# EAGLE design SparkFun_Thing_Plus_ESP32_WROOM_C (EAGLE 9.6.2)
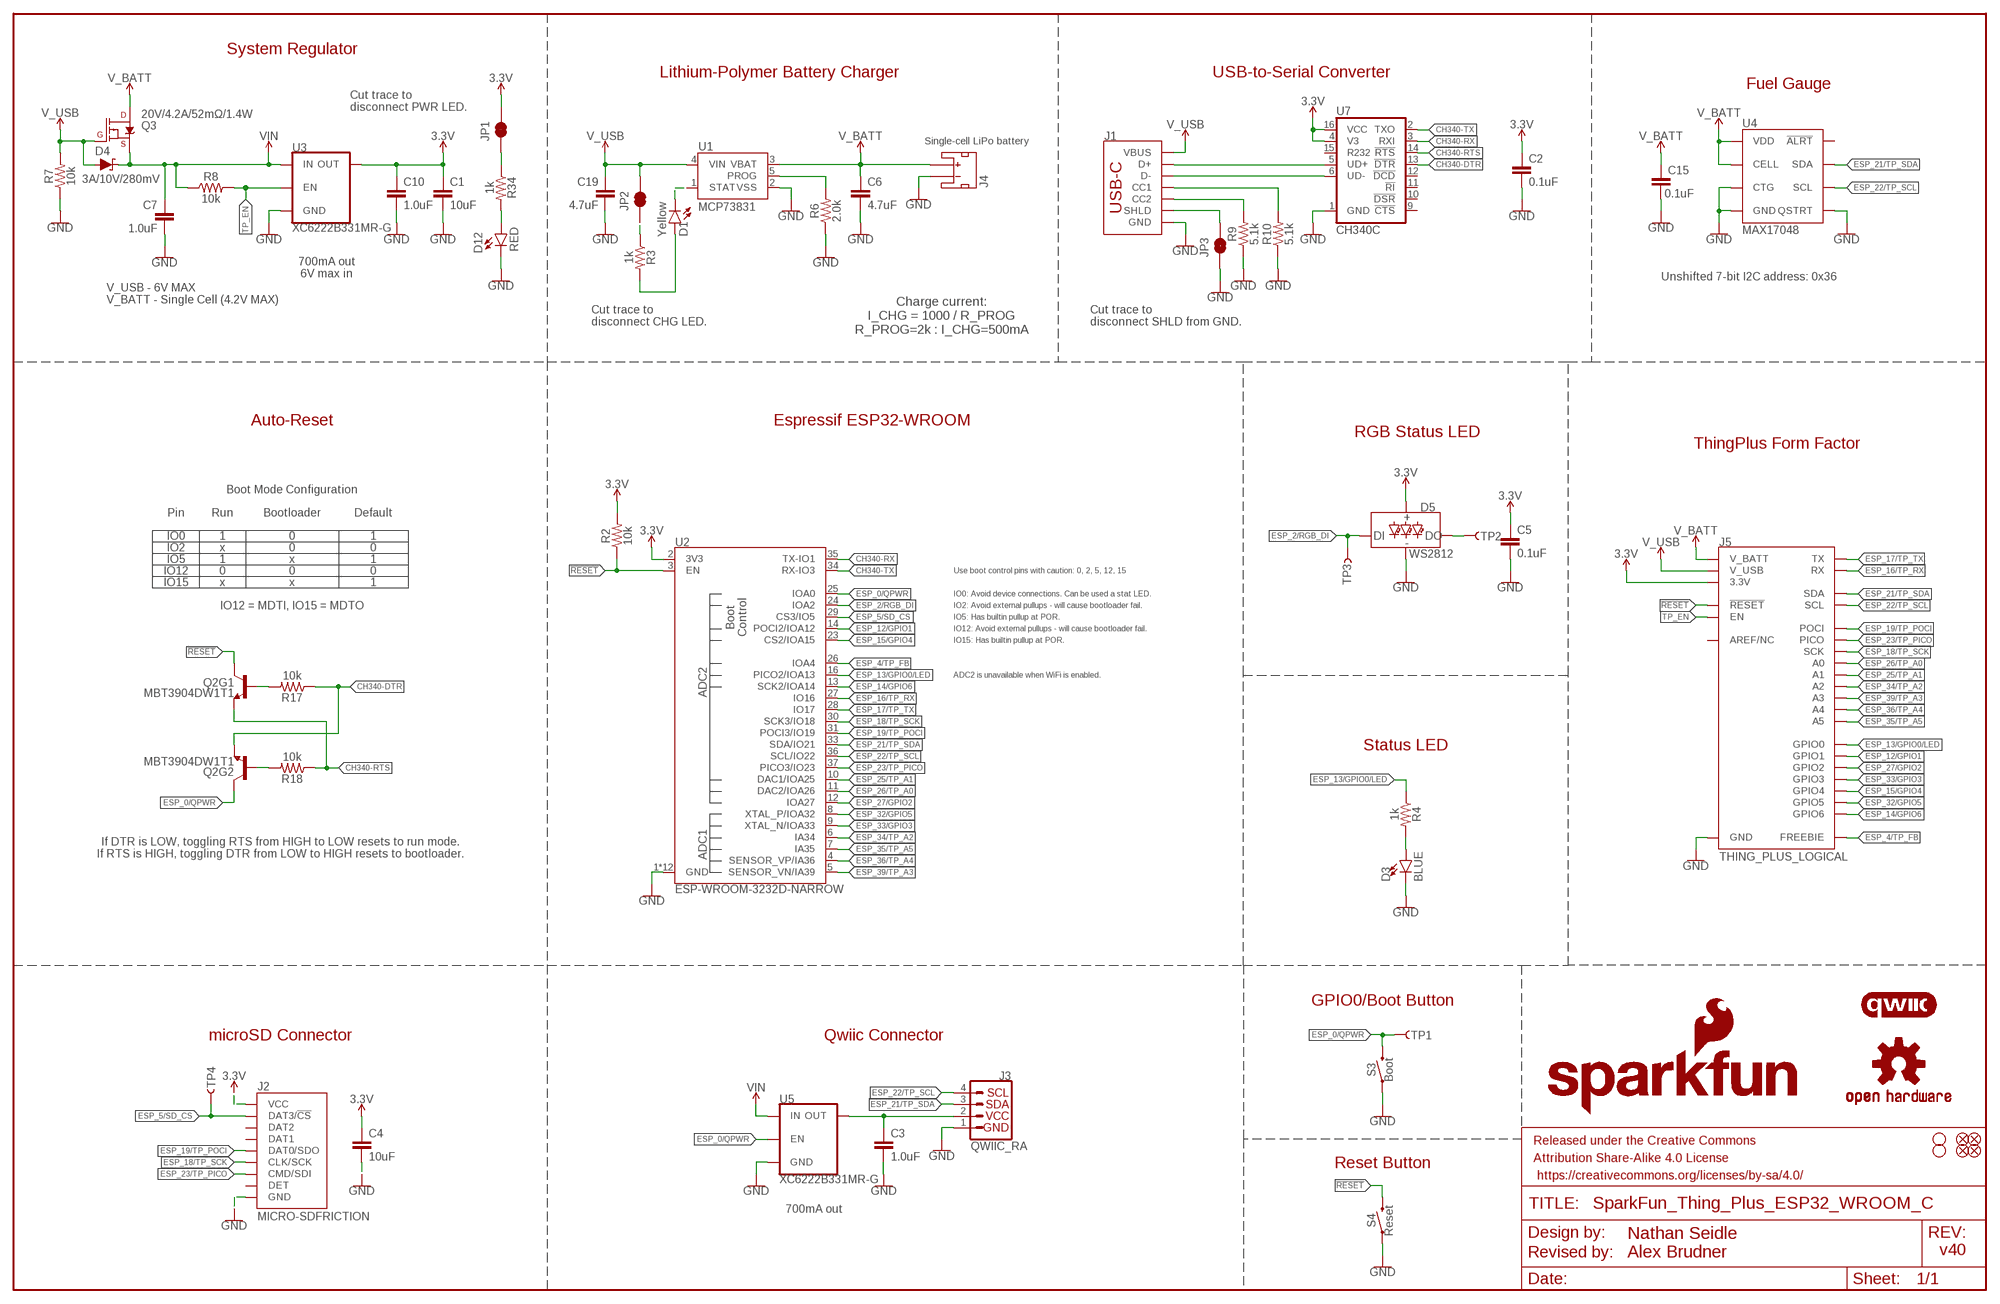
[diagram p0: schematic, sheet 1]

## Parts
C1  10uF  10UF-0402T-6.3V-20%  [0402-TIGHT]
C2  0.1uF  0.1UF-0402T-6.3V-10%-X7R  [0402-TIGHT]
C3  1.0uF  1.0UF-0402T-16V-10%  [0402-TIGHT]
C4  10uF  10UF-0402T-6.3V-20%  [0402-TIGHT]
C5  0.1uF  0.1UF-0402T-6.3V-10%-X7R  [0402-TIGHT]
C6  4.7uF  4.7UF-0402_TIGHT-6.3V-20%-X5R  [0402-TIGHT]
C7  1.0uF  1.0UF-0402T-16V-10%  [0402-TIGHT]
C10  1.0uF  1.0UF-0402T-16V-10%  [0402-TIGHT]
C15  0.1uF  0.1UF-0402T-16V-10%  [0402-TIGHT]
C19  4.7uF  4.7UF-0603-35V-(20%)  [0603]
D1  Yellow  LED-YELLOW0603  [LED-0603]
D3  BLUE  LED-BLUE0603  [LED-0603]
D4  3A/10V/280mV  DIODE-SCHOTTKY-BAT60A  [SOD-323]
D5  WS2812  WS2812_2020  [WS2812-2020]
D12  RED  LED-RED0603  [LED-0603]
FD1  FIDUCIALUFIDUCIAL  [FIDUCIAL-MICRO]
FD2  FIDUCIALUFIDUCIAL  [FIDUCIAL-MICRO]
FD3  FIDUCIALUFIDUCIAL  [FIDUCIAL-MICRO]
FD4  FIDUCIALUFIDUCIAL  [FIDUCIAL-MICRO]
FRAME1  FRAME-LEDGER  [CREATIVE_COMMONS]
H1  STAND-OFFTIGHT  [STAND-OFF-TIGHT]
H2  STAND-OFFTIGHT  [STAND-OFF-TIGHT]
J1  USB_C_2-LAYER_PADS  [USB-C-16P-2LAYER-PADS]
J2  MICRO-SDFRICTION  [MICROSD_TINY]
J3  QWIIC_RA  QWIIC_CONNECTORJS-1MM  [JST04_1MM_RA]
J4  JST_2MM_MALE  [JST-2-SMD]
J5  THING_PLUS_LOGICAL  [THING_PLUS]
JP1  JUMPER-SMT_2_NC_TRACE_SILK  [SMT-JUMPER_2_NC_TRACE_SILK]
JP2  JUMPER-SMT_2_NC_TRACE_SILK  [SMT-JUMPER_2_NC_TRACE_SILK]
JP3  JUMPER-SMT_2_NC_TRACE_SILK  [SMT-JUMPER_2_NC_TRACE_SILK]
LOGO1  SFE_LOGO_NAME_FLAME.1_INCH  [SFE_LOGO_NAME_FLAME_.1]
LOGO2  OSHW-LOGOMINI  [OSHW-LOGO-MINI]
LOGO4  QWIIC_LOGO_4MM  [QWIIC_4MM]
Q2  MBT3904DW1T1  TRANS_NPN_DUAL-MBT3904DW1T1  [SC70-6]
Q3  20V/4.2A/52mΩ/1.4W  MOSFET_PCH-DMG2305UX-7  [SOT23-3]
R2  10k  10KOHM-0402T-1/16W-1%  [0402-TIGHT]
R3  1k  1KOHM-0402T-1/16W-1%  [0402-TIGHT]
R4  1k  1KOHM-0402T-1/16W-1%  [0402-TIGHT]
R6  2.0k  2.0KOHM-0603-1/10W-5%  [0603]
R7  10k  10KOHM-0402T-1/16W-1%  [0402-TIGHT]
R8  10k  10KOHM-0402T-1/16W-1%  [0402-TIGHT]
R9  5.1k  5.1KOHM-0402T-1/16W-1%  [0402-TIGHT]
R10  5.1k  5.1KOHM-0402T-1/16W-1%  [0402-TIGHT]
R17  10k  10KOHM-0402T-1/16W-1%  [0402-TIGHT]
R18  10k  10KOHM-0402T-1/16W-1%  [0402-TIGHT]
R34  1k  1KOHM-0402T-1/16W-1%  [0402-TIGHT]
S3  Boot  MOMENTARY-SWITCH-SPST-SMD-4.6X2.8MM  [TACTILE_SWITCH_SMD_4.6X2.8MM]
S4  Reset  MOMENTARY-SWITCH-SPST-SMD-4.6X2.8MM  [TACTILE_SWITCH_SMD_4.6X2.8MM]
TP1  TEST-POINT3X5  [PAD.03X.05]
TP2  TEST-POINT3X5  [PAD.03X.05]
TP3  TEST-POINT3X5  [PAD.03X.05]
TP4  TEST-POINT3X5  [PAD.03X.05]
U1  MCP73831  [SOT23-5]
U2  ESP-WROOM-3232D-NARROW  [ESP-WROOM-32D-NARROW]
U3  XC6222B331MR-G  [SOT23-5]
U4  MAX17048  MAX17048DFN8  [DFN-8]
U5  XC6222B331MR-G  [SOT23-5]
U7  CH340C  [SO016]

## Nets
3.3V [power]: C1.1 C2.1 C4.1 C5.1 C10.1 D5.VCC J2.4(VCC) J5.27(3.3V) JP1.2 R2.2 U2.2(3V3) U3.5(OUT) U7.4(V3) U7.16(VCC)
!RESET!: J5.28(!RESET) Q2.3(C) R2.1 S4.3 S4.4 U2.3(EN)
CH340-DTR: Q2.1(E) R17.1 U7.13(!DTR)
CH340-RTS: Q2.4(E) R18.1 U7.14(!RTS)
CH340-RX: U2.35(TX-IO1) U7.3(RXI)
CH340-TX: U2.34(RX-IO3) U7.2(TXO)
CHG_LED: D1.A R3.2
D+: J1.A6(D+) J1.B6(D+) U7.5(UD+)
D-: J1.A7(D-) J1.B7(D-) U7.6(UD-)
DTR-10K: Q2.5(B) R17.2
ESP_0/QPWR: Q2.6(C) S3.3 S3.4 TP1.1 U2.25(IOA0) U5.3(EN)
ESP_2/RGB_DI: D5.DI TP3.1 U2.24(IOA2)
ESP_4/TP_FB: J5.13(FREEBIE) U2.26(IOA4)
ESP_5/SD_CS: J2.2(DAT3/!CS!) TP4.1 U2.29(CS3/IO5)
ESP_12/GPIO1: J5.8(GPIO1) U2.14(POCI2/IOA12)
ESP_13/GPIO0/LED: J5.9(GPIO0) R4.1 U2.16(PICO2/IOA13)
ESP_14/GPIO6: J5.3(GPIO6) U2.13(SCK2/IOA14)
ESP_15/GPIO4: J5.5(GPIO4) U2.23(CS2/IOA15)
ESP_16/TP_RX: J5.15(RX) U2.27(IO16)
ESP_17/TP_TX: J5.14(TX) U2.28(IO17)
ESP_18/TP_SCK: J2.5(CLK/SCK) J5.18(SCK) U2.30(SCK3/IO18)
ESP_19/TP_POCI: J2.7(DAT0/SDO) J5.16(POCI) U2.31(POCI3/IO19)
ESP_21/TP_SDA: J3.3 J5.1(SDA) U2.33(SDA/IO21) U4.8(SDA)
ESP_22/TP_SCL: J3.4 J5.2(SCL) U2.36(SCL/IO22) U4.7(SCL)
ESP_23/TP_PICO: J2.3(CMD/SDI) J5.17(PICO) U2.37(PICO3/IO23)
ESP_25/TP_A1: J5.23(A1) U2.10(DAC1/IOA25)
ESP_26/TP_A0: J5.24(A0) U2.11(DAC2/IOA26)
ESP_27/GPIO2: J5.7(GPIO2) U2.12(IOA27)
ESP_32/GPIO5: J5.4(GPIO5) U2.8(XTAL_P/IOA32)
ESP_33/GPIO3: J5.6(GPIO3) U2.9(XTAL_N/IOA33)
ESP_34/TP_A2: J5.22(A2) U2.6(IA34)
ESP_35/TP_A5: J5.19(A5) U2.7(IA35)
ESP_36/TP_A4: J5.20(A4) U2.4(SENSOR_VP/IA36)
ESP_39/TP_A3: J5.21(A3) U2.5(SENSOR_VN/IA39)
GND: C1.2 C2.2 C3.2 C4.2 C5.2 C6.2 C7.2 C10.2 C15.2 C19.2 D3.C D5.GND D12.C J1.GND J1.GND2(GND) J2.6(GND) J2.GND1(GND) J2.GND2(GND) J2.GND3(GND) J2.GND4(GND) J2.GND5(GND) J2.GND6(GND) J3.1 J4.1(-) J5.25(GND) JP3.1 R6.1 R7.1 R9.1 R10.1 S3.1 S3.2 S4.1 S4.2 U1.2(VSS) U2.1(GND) U2.15(GND) U2.38(GND) U2.GND1(GND) U2.GNDT1(GND) U2.GNDT2(GND) U2.GNDT3(GND) U2.GNDT4(GND) U2.GNDT5(GND) U2.GNDT6(GND) U2.GNDT7(GND) U2.GNDT8(GND) U3.2(GND) U4.1(CTG) U4.4(GND) U4.6(QSTRT) U4.9(GND) U5.2(GND) U7.1(GND)
N$1: JP1.1 R34.1
N$2: D3.A R4.2
N$3: D5.DO TP2.1
N$4: JP2.1 R3.1
N$5: J1.B5(CC2) R9.2
N$6: J1.A5(CC1) R10.2
N$7: D1.C U1.1(STAT)
N$8: J1.SHLD1(SHLD) J1.SHLD2(SHLD) J1.SHLD3(SHLD) J1.SHLD4(SHLD) JP3.2
N$14: R6.2 U1.5(PROG)
N$30: D12.A R34.2
QWIIC_PWR [power]: C3.1 J3.2 U5.5(OUT)
RTS-10K: Q2.2(B) R18.2
TP_EN: J5.11(EN) R8.2 U3.3(EN)
V_BATT [power]: C6.1 C15.1 J4.2(+) J5.12(V_BATT) Q3.3(D) U1.3(VBAT) U4.2(CELL) U4.3(VDD)
V_USB [power]: C19.1 D4.A J1.VBUS1(VBUS) J1.VBUS2(VBUS) J5.10(V_USB) JP2.2 Q3.1(G) R7.2 U1.4(VIN)
VIN [power]: C7.1 D4.C Q3.2(S) R8.1 U3.1(IN) U5.1(IN)
Unconnected: J2.1(DAT2) J2.8(DAT1) J2.9(DET) J4.NC1(PAD1) J4.NC2(PAD2) J5.26(AREF/NC) U4.5(!ALRT) U7.9(!CTS) U7.10(!DSR) U7.11(!RI) U7.12(!DCD) U7.15(R232)

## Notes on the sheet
- System Regulator
- Lithium-Polymer Battery Charger | USB-to-Serial Converter
- Fuel Gauge
- Cut trace to 
  disconnect PWR LED.
- Single-cell LiPo battery
- 700mA out
  6V max in
- Unshifted 7-bit I2C address: 0x36
- V_USB - 6V MAX
  V_BATT - Single Cell (4.2V MAX)
- Charge current:
  I_CHG = 1000 / R_PROG
  R_PROG=2k : I_CHG=500mA
- Cut trace to 
  disconnect CHG LED.
- Cut trace to 
  disconnect SHLD from GND.
- Auto-Reset | Espressif ESP32-WROOM
- RGB Status LED
- ThingPlus Form Factor
- Boot Mode Configuration
- Pin | Run | Bootloader | Default
- IO0 | 1 | 0 | 1
- IO2 | x | 0 | 0
- IO5 | 1 | x | 1
- IO12 | 0 | 0 | 0 | Use boot control pins with caution: 0, 2, 5, 12, 15
- IO15 | x | x | 1
- IO0: Avoid device connections. Can be used a stat LED.
- IO12 = MDTI, IO15 = MDTO | IO2: Avoid external pullups - will cause bootloader fail.
- IO5: Has builtin pullup at POR.
- IO12: Avoid external pullups - will cause bootloader fail.
- IO15: Has builtin pullup at POR.
- ADC2 is unavailable when WiFi is enabled.
- Status LED
- If DTR is LOW, toggling RTS from HIGH to LOW resets to run mode.
  If RTS is HIGH, toggling DTR from LOW to HIGH resets to bootloader.
- GPIO0/Boot Button
- microSD Connector | Qwiic Connector
- Reset Button
- 700mA out
- v40

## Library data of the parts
C1 C4 = SparkFun-Capacitors:10UF: 10.0µF ceramic capacitors; PROD_ID: CAP-14848
C2 C5 = SparkFun-Capacitors:0.1UF: 0.1µF ceramic capacitors; PROD_ID: CAP-14993
C3 C7 C10 = SparkFun-Capacitors:1.0UF: 1µF ceramic capacitors; PROD_ID: CAP-12417
C6 = SparkFun-Capacitors:4.7UF: 4.7µF ceramic capacitors; PROD_ID: CAP-14240
C15 = SparkFun-Capacitors:0.1UF: 0.1µF ceramic capacitors; PROD_ID: CAP-12416
C19 = SparkFun-Capacitors:4.7UF: 4.7µF ceramic capacitors; PROD_ID: CAP-14106
D1 = SparkFun-LED:LED-YELLOW: Yellow SMD LED; PROD_ID: DIO-09003
D3 = SparkFun-LED:LED-BLUE: Blue SMD LED; PROD_ID: DIO-08575
D4 = SparkFun-DiscreteSemi:DIODE-SCHOTTKY: Schottky diode; PROD_ID: DIO-14072
D5 = SparkFun-LED:WS2812: Addressable RGB LED - 1 Wire Common names: WS2812, SK6812, Neopixel, APA-106, etc. SMD LED with built-in controller IC. Color: Red/Green/Blue SparkFun Products: LED-SMD RGB (WS2812) LED - RGB Addressable, PTH, 5mm Diffused (5 Pack) LED - RGB Addressable, PTH, 5mm Clear (5 Pack) Blynk Board -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; PROD_ID: DIO-15591
D12 = SparkFun-LED:LED-RED: Red SMD LED; PROD_ID: DIO-00819
FD1-FD4 = SparkFun-Aesthetics:FIDUCIAL: Fiducial Alignment Points
FRAME1 = SparkFun-Aesthetics:FRAME-LEDGER: Schematic Frame - Ledger; DESIGNER: Nathan Seidle; REV_BY: Revised by:; REV_DES: Alex Brudner
H1 H2 = SparkFun-Hardware:STAND-OFF: Stand Off
J1 = SparkFun-Connectors:USB_C: USB Type C 16Pin Connector Super Speed pins not available on the 16-pin purely SMD connector so this part is best for USB 2.0 implementations. D1 and D2 are tied together enabling D+/- no matter which way the cable is plugged into the connector. The two channel configuration pins (CC1/2) are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; PROD_ID: CONN-14122
J2 = SparkFun-Connectors:MICRO-SD: microSD Socket for Transflash Various sockets for µSD. tDoc lines correctly indicate media card edge positions when inserting (unlocked, locked, depressed). NOTE: CD1 and CD2 are connected internally, and the default detect state of the socket is detect pin to ground. SparkFun Products: WAV Trigger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; PROD_ID: CONN-13500
J3 = SparkFun-Connectors:QWIIC_CONNECTOR: SparkFun I2C Standard Qwiic Connector An SMD 1mm pitch JST connector makes it easy and quick (get it? Qwiic?) to connect I2C devices to each other. The Qwiic system enables fast and solderless connection between popular platforms and various sensors and actuators. We carry 200mm, 100mm, 50mm, and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; PROD_ID: CONN-13694; VALUE: QWIIC_RIGHT_ANGLE
J4 = SparkFun-Connectors:JST_2MM_MALE: JST 2MM MALE RA CONNECTOR Two pin, compact surface mount connector. Commonly used as a battery input connection point. We really like the solid locking feeling and high current rating on these small connectors. We use these all the time as battery connectors. Mates to single-cell LiPo batteries.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; PROD_ID: CONN-11443; SF_ID: PRT-08612
J5 = SparkFun-Boards:THING_PLUS_LOGICAL
JP1-JP3 = SparkFun-Jumpers:JUMPER-SMT_2_NC_TRACE: Normally closed trace jumper
LOGO1 = SparkFun-Aesthetics:SFE_LOGO_NAME_FLAME: SparkFun Font Logo w/ Flame
LOGO2 = SparkFun-Aesthetics:OSHW-LOGO: Open-Source Hardware (OSHW) Logo
LOGO4 = SparkFun-Aesthetics:QWIIC_LOGO: Qwiic Logos for placement on schematic and PCB. The 5.5mm silk logo is best for placing next to Qwiic connector.
Q2 = SparkFun-DiscreteSemi:TRANS_NPN_DUAL: Dual NPN Transistors in Single Package The MBT3904W1 puts two general purpose 3904 NPN transistors in a single package. Datasheet SparkFun Products: SparkFun ESP32 Thing; PROD_ID: TRANS-13337
Q3 = SparkFun-DiscreteSemi:MOSFET_PCH: P-channel MOSFETs Voltage controlled devices that allow control of high current outputs. SparkFun Products: SparkFun ESP32 Thing SparkFun ESP8266 Thing SparkFun Pi Servo HAT V2 DMG2305UX-7 (20V/4.2A/SOT23-3); PROD_ID: TRANS-14388
R2 R7 R8 R17 R18 = SparkFun-Resistors:10KOHM: 10kΩ resistor; PROD_ID: RES-14241
R3 R4 R34 = SparkFun-Resistors:1KOHM: 1kΩ resistor; PROD_ID: RES-14342
R6 = SparkFun-Resistors:2.0KOHM: 2kΩ resistor; PROD_ID: RES-08296
R9 R10 = SparkFun-Resistors:5.1KOHM; PROD_ID: RES-14340
S3 S4 = SparkFun-Switches:MOMENTARY-SWITCH-SPST: Momentary Switch (Pushbutton) - SPST; PROD_ID: SWCH-15606
TP1-TP4 = SparkFun-Connectors:TEST-POINT: SparkFun Test Points
U1 = SparkFun-IC-Power:MCP73831: MCP73831T Li-Ion, Li-Pol Controller Miniature single cell, fully integrated Li-Ion, Li-polymer charge management controller Datasheet SparkFun Products: SparkFun ESP32 Thing SparkFun 9DoF Razor IMU M0; PROD_ID: IC-09995
U2 = SparkFun-RF:ESP-WROOM-32: ESP-WROOM-32D - trace antenna (includes keepout) ESP-WROOM-32U - U.FL antenna connector Includes both "standard" footprints and "narrow" version (for use with tighter layouts).; PROD_ID: IC-15676
U3 U5 = SparkFun-IC-Power:XC6222; IOUT: 700mA; PROD_ID: VREG-16775; VOUT: 3.3V
U4 = SparkFun-IC-Power:MAX17048: Micropower 1-Cell Li+ ModelGauge SparkFun Products Qduino Mini (DEV-13614); PROD_ID: IC-12551
U7 = SparkFun-IC-Comms:CH340C; PROD_ID: IC-14038

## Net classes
0 default: width 0.127 mm, drill 0.305 mm
1 power: width 0.305 mm, drill 0.305 mm

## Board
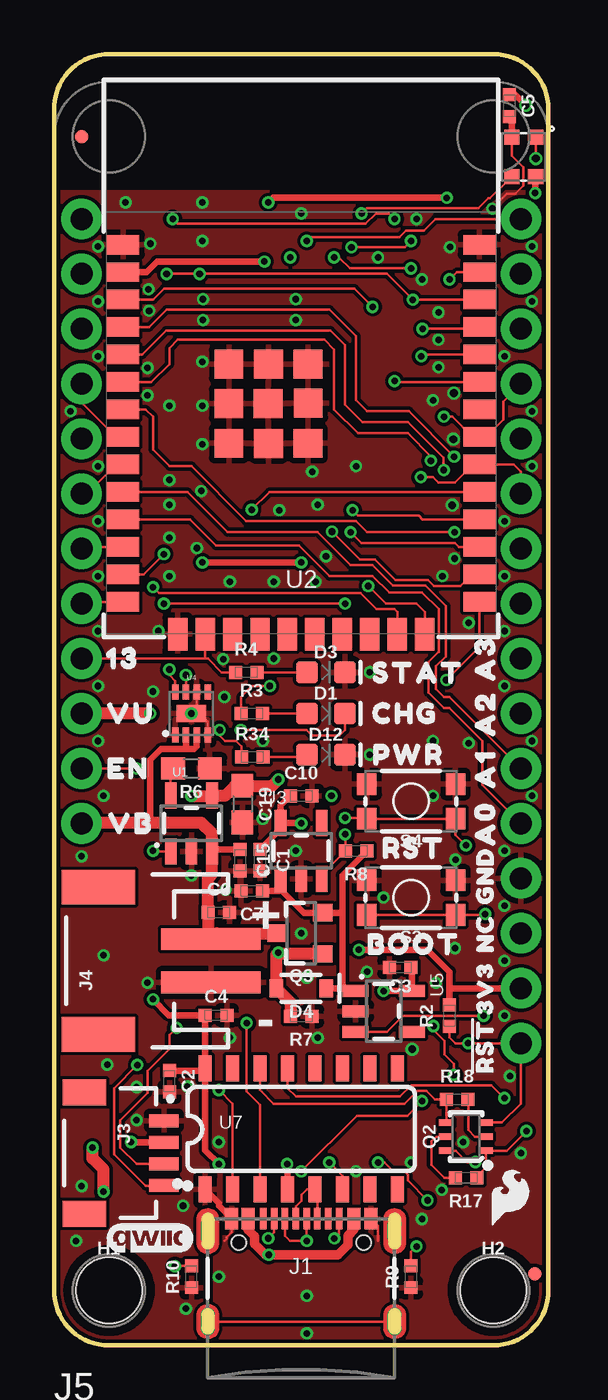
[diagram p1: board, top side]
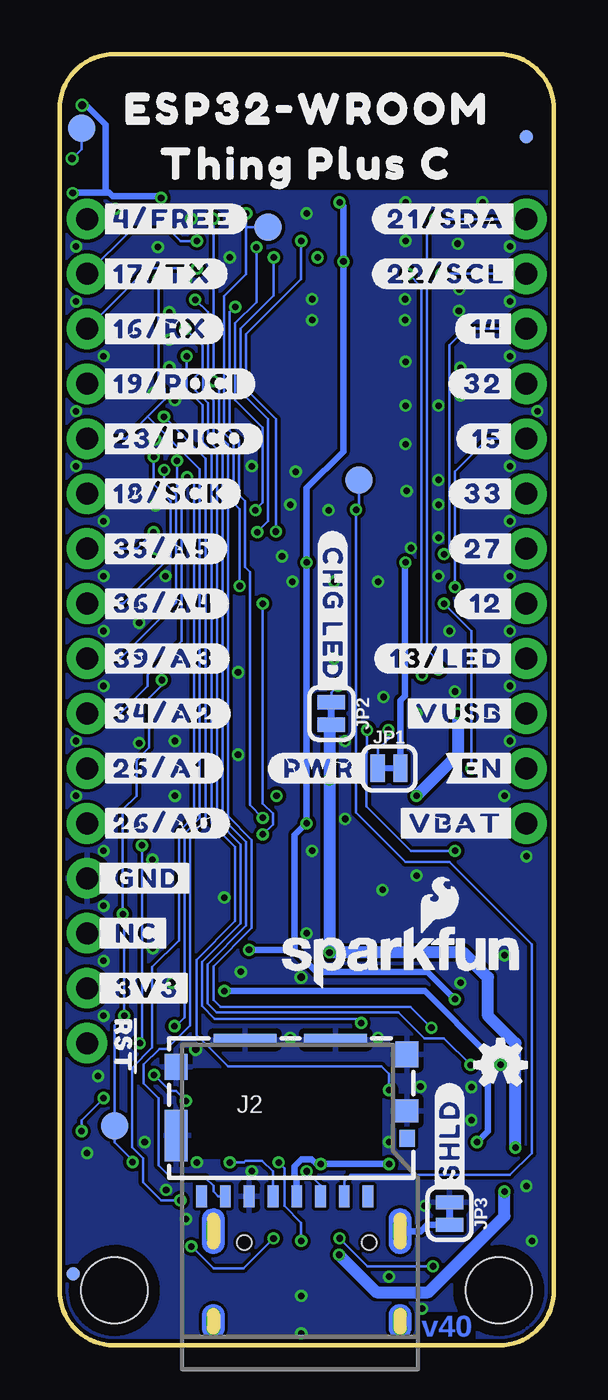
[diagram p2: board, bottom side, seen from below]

Size 22.86 x 59.69 mm. Coordinates in mm from the lower left corner, seen from the top.
Outline: 22.86,2.54 22.86,57.15 arc90 20.32,59.69 2.54,59.69 arc90 0,57.15 0,2.54 arc90 2.54,0 20.32,0 arc90 22.86,2.54
Copper layers (1*16): Top/Horz 0.035mm / dielectric 1.5mm / Bottom/Vert 0.035mm
Design rules "SparkFun-2-Layer-Minimum-JLCPCB": minimum track width 5mil, minimum drill 0.3mm, track to track 5mil, track to pad 5mil, pad to pad 5mil, via to via 5mil, smd to smd 5mil, copper to edge 7mil, drill to drill 7mil, minimum pad ring 5mil, minimum via ring 5mil, stop-mask expansion 4mil, vias tented up to drill 25mil, thermal gap 10mil
tRestrict: area 6.2,26.5 to 6.4,27; area 7.8,23.9 to 8,24.4

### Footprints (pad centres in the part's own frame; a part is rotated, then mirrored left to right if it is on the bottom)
0402-TIGHT = smd 0.6 x 0.6: 1 -0.5,0; 2 0.5,0
0603 = smd 1.1 x 1: 1 -0.85,0; 2 0.85,0
LED-0603 = smd 1 x 1: A -0.877,0; C 0.877,0
SOD-323 = smd 0.63 x 0.83: A 1.15,0; C -1.15,0
WS2812-2020 = smd 0.7 x 0.7: DI -0.915,0.55; DO 0.915,-0.55; GND 0.915,0.55; VCC -0.915,-0.55
FIDUCIAL-MICRO = smd 0.635 x 0.635: 1 0,0
STAND-OFF-TIGHT = hole 3.048: 0,0
USB-C-16P-2LAYER-PADS = smd 0.3 x 1: A5 -1.25,-0.34; A6 -0.25,-0.34; A7 0.25,-0.34; A8 1.25,-0.34; B5 1.75,-0.34; B6 0.75,-0.34; B7 -0.75,-0.34; B8 -1.75,-0.34 | smd 0.6 x 1: GND -3.225,-0.34; GND2 3.225,-0.34; VBUS1 -2.45,-0.34; VBUS2 2.45,-0.34 | drill 0.4 pad 0.6 long: SHLD1 -4.318,-0.915; SHLD2 4.318,-0.915; SHLD3 -4.318,-5.095; SHLD4 4.318,-5.095 | hole 0.65: -2.89,-1.445; 2.89,-1.445
MICROSD_TINY = smd 0.5 x 1: 1 3.55,-3.85; 2 2.45,-3.85; 3 1.35,-3.85; 4 0.25,-3.85; 5 -0.85,-3.85; 6 -1.95,-3.85; 7 -3.05,-3.85; 8 -4.15,-3.85 | smd 0.72 x 0.78: 9 5.35,-1.17 | smd 1.05 x 1.08: GND1 5.35,0.1 | smd 1.05 x 1.2: GND2 5.35,2.71; GND3 -5.325,2.14 | smd 1.05 x 2.39: GND4 -5.325,-1.045 | smd 2.91 x 0.55: GND5 -2.145,3.385; GND6 2.045,3.385
JST04_1MM_RA = smd 0.6 x 1.35: 1 -1.5,0; 2 -0.5,0; 3 0.5,0; 4 1.5,0 | smd 1.2 x 2: NC1 2.8,-3.675; NC2 -2.8,-3.675
JST-2-SMD = smd 1 x 4.6: 1 -1,-3.7; 2 1,-3.7 | smd 1.6 x 3.4: NC1 -3.4,1.5; NC2 3.4,1.5
THING_PLUS = drill 1.016 pad 1.88: 1 1.27,52.07; 2 1.27,49.53; 3 1.27,46.99; 4 1.27,44.45; 5 1.27,41.91; 6 1.27,39.37; 7 1.27,36.83; 8 1.27,34.29; 9 1.27,31.75; 10 1.27,29.21; 11 1.27,26.67; 12 1.27,24.13; 13 21.59,52.07; 14 21.59,49.53; 15 21.59,46.99; 16 21.59,44.45; 17 21.59,41.91; 18 21.59,39.37; 19 21.59,36.83; 20 21.59,34.29; 21 21.59,31.75; 22 21.59,29.21; 23 21.59,26.67; 24 21.59,24.13; 25 21.59,21.59; 26 21.59,19.05; 27 21.59,16.51; 28 21.59,13.97
SMT-JUMPER_2_NC_TRACE_SILK = smd 0.66 x 1.27: 1 -0.521,0; 2 0.521,0
SC70-6 = smd 0.3 x 0.66: 1 -0.65,-0.92; 2 0,-0.92; 3 0.65,-0.92; 4 0.65,0.92; 5 0,0.92; 6 -0.65,0.92
SOT23-3 = smd 0.8 x 0.9: 1 -0.95,-1; 2 0.95,-1; 3 0,1.1
TACTILE_SWITCH_SMD_4.6X2.8MM = smd 0.9 x 1: 1 -2.05,-0.8; 2 2.05,-0.8; 3 2.05,0.8; 4 -2.05,0.8
PAD.03X.05 = smd 1.27 x 1.27: 1 0,0
SOT23-5 = smd 0.55 x 1.2: 1 -0.95,-1.3; 2 0,-1.3; 3 0.95,-1.3; 4 0.95,1.3; 5 -0.95,1.3
ESP-WROOM-32D-NARROW = smd 0.9 x 1.5: 1 6.43,8.238; 2 5.16,8.238; 3 3.89,8.238; 4 2.62,8.238; 5 1.35,8.238; 6 0.08,8.238; 7 -1.19,8.238; 8 -2.46,8.238; 9 -3.73,8.238; 10 -5,8.238; 11 -6.27,8.238; 12 -7.54,8.238; 13 -8.81,8.238; 14 -10.08,8.238; 25 -10.08,-8.238; 26 -8.81,-8.238; 27 -7.54,-8.238; 28 -6.27,-8.238; 29 -5,-8.238; 30 -3.73,-8.238; 31 -2.46,-8.238; 32 -1.19,-8.238; 33 0.08,-8.238; 34 1.35,-8.238; 35 2.62,-8.238; 36 3.89,-8.238; 37 5.16,-8.238; 38 6.43,-8.238 | smd 1.5 x 0.9: 15 -11.57,5.715; 16 -11.57,4.445; 17 -11.57,3.175; 18 -11.57,1.905; 19 -11.57,0.635; 20 -11.57,-0.635; 21 -11.57,-1.905; 22 -11.57,-3.175; 23 -11.57,-4.445; 24 -11.57,-5.715 | smd 1.33 x 1.33: GND1 -0.912,1.531; GNDT1 -2.751,3.346; GNDT2 -2.761,1.516; GNDT3 -2.751,-0.314; GNDT4 -0.891,-0.324; GNDT5 0.909,-0.314; GNDT6 0.909,1.516; GNDT7 0.909,3.346; GNDT8 -0.921,3.346
DFN-8 = smd 0.3 x 0.7: 1 -0.75,-0.99; 2 -0.25,-0.99; 3 0.25,-0.99; 4 0.75,-0.99; 5 0.75,0.99; 6 0.25,0.99; 7 -0.25,0.99; 8 -0.75,0.99 | smd 1.38 x 0.8: 9 0,0
SO016 = smd 0.6 x 1.2: 1 -4.445,-2.8; 2 -3.175,-2.8; 3 -1.905,-2.8; 4 -0.635,-2.8; 5 0.635,-2.8; 6 1.905,-2.8; 7 3.175,-2.8; 8 4.445,-2.8; 9 4.445,2.8; 10 3.175,2.8; 11 1.905,2.8; 12 0.635,2.8; 13 -0.635,2.8; 14 -1.905,2.8; 15 -3.175,2.8; 16 -4.445,2.8

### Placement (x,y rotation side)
C1  9.53,22.43 270 top
C2  5.33,12.22 270 top
C3  16,17.48 180 top
C4  7.49,15.27 0 top
C5  21.06,57.3 270 top
C6  7.62,20.02 0 top
C7  9.14,21.01 180 top
C10  11.43,25.4 0 top
C15  8.61,22.43 270 top
C19  8.71,25.02 270 top
D1  12.57,29.21 0 top
D3  12.57,31.11 0 top
D4  11.43,16.51 180 top
D5  21.72,54.94 90 top
D12  12.57,27.3 0 top
FD1  1.27,55.88 0 top
FD2  1.27,55.88 0 bottom
FD3  22.23,3.3 0 top
FD4  22.23,3.3 0 bottom
FRAME1  not placed on the board
H1  2.54,2.54 0 top
H2  20.32,2.54 0 top
J1  11.43,6.2 0 top
J2  12.14,10.74 0 bottom
J3  5.08,8.89 270 top
J4  3.56,17.78 90 top
J5  0,0 0 top
JP1  7.62,26.67 0 bottom
JP2  10.29,29.21 270 bottom
JP3  4.83,6.1 270 bottom
LOGO1  7.01,17.96 0 bottom
LOGO2  2.46,12.98 0 bottom
LOGO4  4.45,4.95 0 top
Q2  19.05,9.65 90 top
Q3  11.43,19.05 90 top
R2  18.29,15.24 90 top
R3  9.14,29.21 0 top
R4  8.89,31.11 0 top
R6  6.35,26.67 180 top
R7  11.43,15.21 180 top
R8  13.97,22.86 180 top
R9  16.51,3.17 90 top
R10  6.35,3.17 90 top
R17  19.05,7.75 180 top
R18  18.64,11.38 0 top
R34  9.17,27.2 0 top
S3  16.51,20.7 180 top
S4  16.51,25.15 180 top
TP1  20.32,10.16 0 bottom
TP2  21.84,56.26 0 bottom
TP3  13.21,51.69 0 bottom
TP4  9.02,40.01 0 bottom
U1  6.35,24.13 0 top
U2  11.43,44.45 90 top
U3  11.43,22.86 0 top
U4  6.35,29.21 0 top
U5  15.24,15.44 270 top
U7  11.43,10.01 0 top
U$1  [SFE_LOGO_FLAME_STOP_.1]  21.34,6.86 0 bottom
U$2  [#23#PICO#0]  21.08,41.91 0 bottom
U$3  [#19#POCI#0]  21.08,44.45 0 bottom
U$4  [#4#FREE#0]  21.08,52.07 0 bottom
U$5  [#CHG_LED#0]  10.24,37.62 270 bottom
U$6  [ESP32#WROOM0]  11.43,57.15 0 bottom
U$7  [THING_PLUS_C0]  11.43,54.61 0 bottom
U$8  [#SHLD#0]  4.83,6.93 90 bottom
U$9  [#_GND#0]  21.34,21.59 0 bottom
U$10  [#_NC#0]  21.34,19.05 0 bottom
U$11  [#_3V3#0]  21.34,16.51 0 bottom
U$12  [SFE_LOGO_FLAME_.1]  21.08,6.86 0 top
U$23  [3V30]  19.94,16.51 90 top
U$24  [CHG1]  16.23,29.21 0 top
U$25  [PWR2]  16.38,27.3 0 top
U$26  [STAT0]  16.84,31.09 0 top
U$68  [A03]  19.94,24.13 90 top
U$69  [A12]  19.94,26.67 90 top
U$70  [A21]  19.94,29.21 90 top
U$71  [A30]  19.94,31.75 90 top
U$72  [#17#TX#0]  21.08,49.53 0 bottom
U$73  [VB1]  3.56,24.13 0 top
U$74  [EN3]  3.43,26.67 0 top
U$75  [GND1]  19.94,21.72 90 top
U$76  [VU0]  3.56,29.21 0 top
U$77  [130]  3.17,31.75 0 top
U$78  [BOOT0]  16.64,18.54 0 top
U$79  [#RST#0]  19.81,13.84 90 top
U$80  [RST0]  16.64,22.99 0 top
U$81  [#16#RX#0]  21.08,46.99 0 bottom
U$83  [#18#SCK#0]  21.08,39.37 0 bottom
U$84  [#35#A5#0]  21.08,36.83 0 bottom
U$85  [#36#A4#0]  21.08,34.29 0 bottom
U$86  [#25#A1#2]  21.08,26.67 0 bottom
U$87  [#26#A0#3]  21.08,24.13 0 bottom
U$88  [#34#A2#1]  21.08,29.21 0 bottom
U$89  [#39#A3#0]  21.08,31.75 0 bottom
U$90  [#12#4]  1.65,34.29 0 bottom
U$91  [#14#9]  1.65,46.99 0 bottom
U$92  [#15#7]  1.65,41.91 0 bottom
U$93  [#27#5]  1.65,36.83 0 bottom
U$94  [#32#8]  1.65,44.45 0 bottom
U$95  [#33#6]  1.65,39.37 0 bottom
U$96  [#EN#1]  1.65,26.67 0 bottom
U$97  [#VBAT#0]  1.65,24.13 0 bottom
U$98  [#VUSB#2]  1.65,29.21 0 bottom
U$99  [#13#LED#0]  1.65,31.75 0 bottom
U$100  [#21#SDA#1]  1.52,52.07 0 bottom
U$101  [#22#SCL#0]  1.52,49.53 0 bottom
U$102  [#PWR#0]  8.51,26.67 0 bottom
U$107  [NC0]  19.94,19.05 90 top
U$109  [#RST#0]  19.81,13.84 270 bottom

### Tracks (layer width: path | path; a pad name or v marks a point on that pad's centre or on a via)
3.3V  (via drill 0.3, 0.35)
  Top/Horz 0.305: v9.73,50.1 4.76,50.1 4.27,49.61 U2.2 | v18.16,53.05 10.12,53.05 v9.91,52.83 | v14.1,18.29 17.27,18.29 18.29,17.27 18.29,16.51 | 6.99,12.7 U7.16 6.99,9.02 v7.62,8.38 | v6.86,36.2 v11.43,36.2 | R2.2 18.29,16.51 | C2.1 5.35,12.7 6.99,12.7 | v4.57,16 5.31,15.27 C4.1 6.99,12.71 6.99,12.7 | v10.78,8.38 10.79,8.37 U7.4 | C10.1 10.48,24.95 U3.5 | U3.5 11.4,24.16 v11.43,24.13 | C5.1 21.34,57.8 v21.81,57.33 | C1.1 10.48,23.88 U3.5 | J5.27 18.29,16.51 | v22.25,53.26 22.25,54.01 D5.VCC
  Bottom/Vert 0.305: v9.91,52.83 9.73,52.65 v9.73,50.1 9.74,50.09 9.74,41.31 11.43,39.62 v11.43,36.2 v11.43,24.13 11.46,24.13 11.99,23.6 11.99,18.29 | v18.16,53.05 18.24,53.12 20.4,53.12 20.56,53.29 20.73,53.29 | JP1.2 7.1,29.82 6.9,30.02 6.9,36.16 v6.86,36.2 | v14.1,18.29 11.99,18.29 | v4.57,16 5.84,17.27 10.97,17.27 11.99,18.29 | v7.62,8.38 v10.78,8.38 10.97,8.38 11.2,8.61 11.66,8.61 11.99,8.28 11.99,7.82 11.89,7.72 J2.4 | v21.81,57.33 21.62,57.33 20.73,56.44 20.73,53.29 | v22.25,53.26 22.12,53.26 22.09,53.29 20.73,53.29
!RESET!  (via drill 0.3)
  Top/Horz 0.127: v19.05,23.11 18.56,23.6 S4.4 S4.3 14.42,24.38 v13.46,24.38 | v14.73,48.01 13.89,48.85 5.1,48.85 4.59,48.34 U2.3 | R2.1 18.29,14.23 18.55,13.97 v19.15,13.97 J5.28 21.59,11.18 20.72,10.3 Q2.3
  Bottom/Vert 0.127: v19.05,23.11 19.05,14.07 v19.15,13.97 | v14.73,48.01 14.99,47.75 14.99,42.28 14.57,41.86 14.57,39.31 14.28,39.02 14.28,35.97 14.06,35.76 14.06,24.98 v13.46,24.38
CH340-DTR  (via drill 0.3)
  Top/Horz 0.127: R17.1 19.55,7.82 19.97,8.24 Q2.1 20.94,9 v21.84,9.91 | U7.13 10.79,11.89 11.18,11.51 16,11.51 16.52,12.02 20.23,12.02 v20.83,11.43
  Bottom/Vert 0.127: v20.83,11.43 21.84,10.41 v21.84,9.91
CH340-RTS
  Top/Horz 0.127: Q2.4 18.14,10.32 R18.1 17.6,11.38 17.21,11.77 16.8,11.77 16.2,11.18 10.16,11.18 9.53,11.81 U7.14
CH340-RX  (via drill 0.3)
  Top/Horz 0.127: U7.3 9.53,11.13 8.91,11.75 v8.91,14.9 | U2.35 19.59,46.99 v17.04,46.99
  Bottom/Vert 0.127: v17.04,46.99 16.26,46.2 16.26,45.09 16.58,44.77 16.57,44.77 16.57,44.13 | v8.91,14.9 9.11,15.1 15.69,15.1 16.27,15.68 16.27,17.72 14.48,19.51 14.48,23.16 15.58,24.26 15.58,41.44 16,41.86 16,43.57 16.57,44.13 | 16.57,44.13 16.58,44.14
CH340-TX  (via drill 0.3)
  Top/Horz 0.127: v16.98,45.72 17.06,45.8 U2.34 | v7.62,11.8 8.26,11.17 U7.2
  Bottom/Vert 0.127: v7.62,11.8 7.62,12.54 7.98,12.9 15.07,12.9 16.53,14.36 16.53,17.83 14.73,19.62 14.73,23.05 15.84,24.16 15.84,41.33 16.26,41.75 16.26,43.46 16.98,44.19 v16.98,45.72
CHG_LED
  Top/Horz 0.127: R3.2 D1.A
D+
  Top/Horz 0.127: J1.A6 11.18,6.42 11.44,6.68 11.44,6.96 11.69,7.21 U7.5 12.18,7.09 J1.B6
D-  (via drill 0.3)
  Top/Horz 0.127: J1.A7 v11.68,4.83 10.92,4.83 10.68,5.07 J1.B7 | v12.72,8.46 13.34,7.85 U7.6
  Bottom/Vert 0.127: v12.72,8.46 12.46,8.19 12.46,6.44 11.68,5.67 v11.68,4.83
DTR-10K
  Top/Horz 0.127: R17.2 18.04,7.75 17.45,8.34 17.45,9.42 17.68,9.65 Q2.5
ESP_0/QPWR  (via drill 0.3)
  Top/Horz 0.127: S3.3 S3.4 19.9,19.9 v19.94,19.94 | U2.25 19.67,32.29 v18.14,30.76 | v19.86,15.24 16.14,15.24 15.4,14.49 U5.3 | Q2.6 18.57,9 19.1,8.47 v19.48,8.47
  Bottom/Vert 0.127: v18.14,30.76 18.14,30.5 18.71,29.93 18.71,27.64 19.3,27.05 19.3,25.4 19.94,24.77 v19.94,19.94 19.86,19.86 v19.86,15.24 20.32,14.78 TP1.1 20.32,9.4 19.48,8.56 v19.48,8.47
ESP_2/RGB_DI  (via drill 0.3)
  Top/Horz 0.127: v14.22,52.32 14.48,52.58 19.63,52.58 20.07,53.02 20.16,53.02 D5.DI | U2.24 17.14,33.91 16.76,34.29 15.34,34.29 v14.53,35.1
  Bottom/Vert 0.127: v14.22,52.32 14.22,51.69 | 14.22,51.69 14.22,49.52 15.24,48.51 15.24,42.17 14.82,41.75 14.82,38.95 14.53,38.66 v14.53,35.1 | TP3.1 14.22,51.69
ESP_4/TP_FB  (via drill 0.3)
  Top/Horz 0.127: v11.68,51.05 11.86,51.23 15.98,51.23 16.27,51.52 17.09,51.52 17.64,52.07 J5.13 | U2.26 19.33,35.64 18.78,35.09 17.57,35.09 17.28,35.38 15.79,35.38 14.83,36.34 14.13,36.34 v12.85,37.62
  Bottom/Vert 0.127: v12.85,37.62 12.85,42.82 14.22,44.2 14.22,46.74 11.68,49.28 v11.68,51.05
ESP_5/SD_CS  (via drill 0.3)
  Top/Horz 0.127: U2.29 9.96,39.45 v9.14,38.63
  Bottom/Vert 0.127: TP4.1 9.02,38.76 v9.14,38.63 9.14,24.64 6.86,22.35 4.83,22.35 1.02,18.54 1.02,8.89 2.03,7.87 9.4,7.87 9.69,7.58 J2.2
ESP_12/GPIO1
  Top/Horz 0.127: J5.8 1.35,34.37 U2.14
ESP_13/GPIO0/LED
  Top/Horz 0.127: R4.1 7.75,31.11 7.11,31.75 6.99,31.75 | U2.16 6.99,31.75 | 6.99,31.75 J5.9
ESP_14/GPIO6  (via drill 0.3)
  Top/Horz 0.127: U2.13 4.14,35.64 v5.08,36.58
  Bottom/Vert 0.127: v5.08,36.58 4.83,36.83 4.83,46.23 4.06,46.99 J5.3
ESP_15/GPIO4  (via drill 0.3)
  Top/Horz 0.127: U2.23 15.88,33.91 15.75,34.04 14.91,34.04 14.17,34.77 4.85,34.77 v4.57,35.05
  Bottom/Vert 0.127: v4.57,35.05 4.57,40.39 3.05,41.91 J5.5
ESP_16/TP_RX  (via drill 0.3)
  Top/Horz 0.127: v16.51,49.78 13.69,49.78 13.21,50.27 12.98,50.27 v12.95,50.29 | v13.72,37.59 14.22,37.08 18.54,37.08 18.72,36.91 U2.27
  Bottom/Vert 0.127: v16.51,49.78 18.8,49.78 J5.15 | v12.95,50.29 12.95,48.51 14.48,46.99 14.48,44.09 13.21,42.82 13.21,38.1 v13.72,37.59
ESP_17/TP_TX  (via drill 0.3)
  Top/Horz 0.127: v16.51,51.05 | v16.51,51.05 16.22,50.76 v13.75,50.76 | v13.8,38.61 14.06,38.35 16.87,38.35 17.04,38.18 U2.28
  Bottom/Vert 0.127: v16.51,51.05 17.27,51.05 17.78,51.56 19.56,51.56 J5.14 | v13.75,50.76 13.75,48.22 14.73,47.24 14.73,43.69 13.46,42.42 13.46,38.95 v13.8,38.61
ESP_18/TP_SCK  (via drill 0.3)
  Top/Horz 0.127: v16.96,40.13 17.53,40.13 17.78,39.88 18.54,39.88 19.38,40.72 U2.30 21.26,40.72 21.59,40.39 J5.18 | v17.27,6.71 16.37,7.62 16.37,7.89 16.15,8.1 15.65,8.1 15.29,8.46 v14.99,8.46
  Bottom/Vert 0.127: J2.5 12.99,8.04 13.49,8.53 14.25,8.53 14.33,8.46 v14.99,8.46 | v17.27,6.71 18.16,6.71 19,7.54 19,8.65 19.49,9.15 19.49,12.84 18.57,13.77 18.57,17.5 17.34,18.73 17.34,23.77 16.63,24.47 16.63,39.81 v16.96,40.13
ESP_19/TP_POCI  (via drill 0.3)
  Top/Horz 0.127: v18.03,42.93 18.41,42.93 19.35,41.99 U2.31 19.97,41.99 20.78,42.8 20.78,43.64 J5.16
  Bottom/Vert 0.127: v18.03,42.93 16.1,40.99 16.1,24.29 16.83,23.55 16.83,14.79 17.91,13.72 18.24,13.72 18.97,12.98 18.97,12.12 18.29,11.43 18.29,8.33 17.7,7.75 16.12,7.75 15.75,7.37 15.75,7.11 15.53,6.89 J2.7
ESP_21/TP_SDA  (via drill 0.3)
  Top/Horz 0.127: v15.75,44.58 15.79,44.53 U2.33 | v15.75,52.07 15.49,52.32 14.89,52.32 14.41,51.84 5.71,51.84 v5.49,52.07 | J3.3 3.81,8.38 3.05,9.14 3.05,10.41 4.32,11.68 4.32,12.7 5.33,13.72 5.33,14.35 v5.66,14.68 | U4.8 5.6,30.72 5.33,30.99 v5.33,31.24
  Bottom/Vert 0.127: v15.75,52.07 v15.75,44.58 15.49,44.32 15.49,42.07 15.07,41.65 15.07,24.47 13.97,23.37 13.97,19.3 15.75,17.53 15.75,15.97 15.42,15.65 6.63,15.65 v5.66,14.68 | v5.33,31.24 5.33,31.62 5.87,32.16 5.87,51.69 v5.49,52.07 J5.1
ESP_22/TP_SCL  (via drill 0.3)
  Top/Horz 0.127: U4.7 v6.1,30.98 v6.1,30.99 | v5.21,49.53 v6.73,49.53 15.39,49.53 v16.59,48.34 U2.36 | J3.4 5.06,7.37 4.24,7.37 2.77,8.84 2.77,11.88 v3.85,12.96
  Bottom/Vert 0.127: v6.1,30.99 6.12,31.01 6.12,48.92 v6.73,49.53 | v3.85,12.96 5.08,14.2 5.99,14.2 7.18,15.39 15.6,15.39 16.02,15.8 16.02,17.61 14.22,19.41 14.22,23.26 15.33,24.37 15.33,41.54 15.75,41.96 15.75,43.67 16.22,44.14 16.22,44.77 16,44.99 16,47.75 v16.59,48.34 | v5.21,49.53 J5.2
ESP_23/TP_PICO  (via drill 0.3)
  Top/Horz 0.127: v17.02,11.3 16.33,10.62 14,10.62 v11.43,8.05 | v18.49,12.5 18.49,13.01 18.05,13.44 18.05,14.07 17.55,14.58 v17.55,14.76 | v18.29,49.28 18.62,49.61 U2.37
  Bottom/Vert 0.127: J2.3 10.79,7.41 v11.43,8.05 | v17.02,11.3 17.48,11.76 17.75,11.76 v18.49,12.5 | v17.55,14.76 17.5,14.76 17.09,15.17 17.09,23.66 16.38,24.37 16.38,40.51 18.8,42.93 | 18.8,42.93 19.81,41.91 J5.17 | v18.29,49.28 18.29,44.51 18,44.22 18,43.72 18.8,42.93
ESP_25/TP_A1
  Top/Horz 0.127: U2.10 6.17,39.45 8.03,37.59 12.19,37.59 13.7,36.08 14.73,36.08 15.68,35.13 17.17,35.13 18.12,34.19 18.12,31.85 17.67,31.4 17.67,30.34 18.03,29.97 18.29,29.97 J5.23
ESP_26/TP_A0
  Top/Horz 0.127: U2.11 6.29,38.18 7.49,36.98 11.33,36.98 12.74,35.57 14.72,35.57 15.5,34.8 17.02,34.8 17.79,34.03 17.79,32.05 17.78,32.05 17.32,31.59 17.32,30.18 18.03,29.46 18.29,29.46 19.81,27.94 19.81,25.91 J5.24
ESP_27/GPIO2
  Top/Horz 0.127: J5.7 1.35,36.91 U2.12
ESP_32/GPIO5
  Top/Horz 0.127: U2.8 2.87,41.99 1.27,43.59 J5.4
ESP_33/GPIO3
  Top/Horz 0.127: U2.9 2.87,40.72 1.52,39.37 J5.6
ESP_34/TP_A2  (via drill 0.3)
  Top/Horz 0.127: U2.6 4.5,44.53 5.33,45.36 5.33,46.1 5.71,46.48 12.5,46.48 12.95,46.02 12.95,43.27 14.06,42.16 16.36,42.16 17.43,41.09 v17.43,40.89
  Bottom/Vert 0.127: v17.43,40.89 17.43,39.72 17.22,39.51 17.22,32.56 18.8,30.99 18.8,30.48 20.07,29.21 J5.22
ESP_35/TP_A5  (via drill 0.3)
  Top/Horz 0.127: U2.7 4.24,43.26 4.57,42.93 4.57,41.4 5.33,40.64 6.35,40.64 8.89,38.1 13.97,38.1 14.48,37.59 v18.52,37.59
  Bottom/Vert 0.127: v18.52,37.59 19.28,36.83 J5.19
ESP_36/TP_A4  (via drill 0.3)
  Top/Horz 0.127: U2.4 4.4,47.07 5.21,47.88 12.74,47.88 13.97,46.65 13.97,43.69 14.48,43.18 16.4,43.18 v18.5,41.08
  Bottom/Vert 0.127: v18.5,41.08 18.5,39.81 17.73,39.04 17.73,36.47 19.86,34.34 19.91,34.29 J5.20
ESP_39/TP_A3  (via drill 0.3)
  Top/Horz 0.127: U2.5 4.06,45.8 5.18,46.91 12.78,46.91 13.46,46.23 13.46,43.48 14.27,42.67 16.36,42.67 18.01,41.03 18.01,40.48 v18.02,40.46
  Bottom/Vert 0.127: v18.02,40.46 18.02,39.9 17.48,39.36 17.48,34.34 20.07,31.75 J5.21
GND  (via drill 0.3, 0.35)
  Top/Horz 0.127: U4.6 6.6,29.46 U4.9 6.73,29.21 7.1,28.84 U4.4 | J1.GND2 14.99,5.53 14.99,4.83 | D5.GND 21.17,54.99 21.71,54.45 21.71,53.6 21.34,53.23 20.95,53.23 v20.27,52.55 | J1.GND 8.21,5.22 7.97,4.99 7.97,4.93 7.87,4.83
  Top/Horz 0.305: U7.1 7.62,6.58 7.62,6.44 J1.GND 8.21,5.51 | C5.2 21.17,56.69 D5.GND
  other vias: 4.32,16.76 3.81,10.41 5.97,6.45 6.1,1.7 6.17,11.96 15.24,20.7 18.57,22.45 14.61,27.3 14.61,31.11 19.18,27.84 11.18,22.86 7.92,21.06 6.35,21.72 6.35,29.21 4.83,33.02 18.31,50.77 4.45,50.93 14.48,17.27 11.68,2.29 13.97,8.05 16.51,8.46 12.19,14.22 18.92,9.4 17.65,16.76 18.54,18.36 7.62,3.17 4.37,48.82 4.39,47.83 6.88,48.36 11.18,48.36 6.88,47.4 11.18,47.4 6.86,51.05 22.1,50.8 22.1,48.26 20.83,45.72 22.1,43.18 22.1,40.64 20.83,38.1 20.83,35.56 20.83,33.02 20.83,30.48 22.1,27.94 17.53,27.94 12.09,35.31 10.16,35.31 8.13,35.31 2.03,50.8 2.03,48.26 2.03,45.72 0.76,43.18 2.03,40.64 2.03,38.1 6.81,39.5 6.6,36.86 5.33,35.56 2.03,35.56 2.03,33.02 10.41,38.61 12.19,38.86 12.57,36.47 5.33,38.86 2.03,30.48 2.03,27.94 2.29,25.4 1.27,22.61 2.29,18.03 2.46,12.98 3.81,11.94 1.27,7.37 10.16,31.75 7.82,31.72 7.87,29.97 4.32,45.19 11.43,52.32 6.86,52.83 3.3,52.83 19.18,33.4 13.97,40.64 11.94,40.39 6.86,41.66 17.53,43.69 17.78,45.21 17.78,46.48 17.02,49.28 16.76,52.07 14.99,50.29 6.86,43.43 6.86,45.47 5.33,43.43 5.33,40.01 5.33,37.34 4.57,30.23 11.43,19.05 8.13,14.22 21.08,12.45 21.59,8.89 17.93,7.19 1.02,4.83 17.02,5.84 20.83,15.24 20.83,17.78 20.83,20.32 20.83,22.86 17.53,25.4 22.1,25.4 7.62,9.4 9.65,27.94 11.68,17.02 16.56,13.69 4.32,43.92 18.47,41.88 17.78,47.75 18.41,38.84 18.49,44.02 18.52,36.37 17.96,35.56 9.65,24.33 11.68,0.56
  pour Bottom/Vert (isolate 0.152): 0,0 0,53.34 22.86,53.34 22.86,0
  pour Top/Horz (isolate 0.152): 22.86,0 22.86,53.34 0,53.34 0,0
N$1  (via drill 0.3)
  Top/Horz 0.127: R34.1 8.67,27.69 8.42,27.94 7.91,27.94 7.66,28.19 v7.66,28.45
  Bottom/Vert 0.127: JP1.1 8.14,27.56 7.66,28.04 v7.66,28.45
N$2
  Top/Horz 0.127: R4.2 D3.A
N$3  (via drill 0.35)
  Top/Horz 0.127: 22.28,55.84 v22.28,54.86
  Top/Horz 0.305: D5.DO 22.28,55.84
  Bottom/Vert 0.127: TP2.1 21.84,55.3 v22.28,54.86
N$4  (via drill 0.3)
  Top/Horz 0.127: v9.98,30.48 9.14,30.48 8.64,29.97 R3.1
  Bottom/Vert 0.127: JP2.1 10.29,30.18 v9.98,30.48
N$5  (via drill 0.3)
  Top/Horz 0.127: J1.B5 13.18,5.16 v12.96,4.94 | v16.76,4.57 16.51,4.32 R9.2
  Bottom/Vert 0.127: v12.96,4.94 14.35,3.56 15.75,3.56 v16.76,4.57
N$6  (via drill 0.3)
  Top/Horz 0.127: J1.A5 10.18,5.22 v9.91,4.95 | v5.59,3.66 5.61,3.67 R10.2
  Bottom/Vert 0.127: v9.91,4.95 8.61,3.66 v5.59,3.66
N$7  (via drill 0.3)
  Top/Horz 0.127: U1.1 4.6,22.83 v4.57,22.86 | v8.64,28.45 11.68,28.45 11.94,28.19 13.21,28.19 13.46,28.45 13.46,29.2 D1.C
  Bottom/Vert 0.127: v4.57,22.86 6.6,22.86 8.66,24.92 8.66,27.38 8.64,27.41 v8.64,28.45
N$8
  Top/Horz 0.127: J1.SHLD2 J1.SHLD4 J1.SHLD3 J1.SHLD1
  Bottom/Vert 0.305: JP3.2 5.83,5.58 5.84,5.59 6.15,5.28 J1.SHLD1
N$13  (via drill 0.3)
  other vias: 12.83,25.4
N$14
  Top/Horz 0.127: U1.5 5.4,26.57 R6.2
N$30
  Top/Horz 0.127: R34.2 11.59,27.2 D12.A
N$51  (via drill 0.3)
  other vias: 10.92,50.29
QWIIC_PWR  (via drill 0.3)
  Top/Horz 0.305: v3.56,9.4 J3.2 | C3.1 16.54,17.44 U5.5 15.25,16.39 v15.24,16.38
  Bottom/Vert 0.305: v3.56,9.4 3.05,9.91 3.05,13.46 5.97,16.38 v15.24,16.38
RTS-10K
  Top/Horz 0.127: Q2.2 19.46,9.65 19.15,9.96 19.15,11.37 R18.2
TP_EN  (via drill 0.3)
  Top/Horz 0.127: v13.46,23.62 v13.47,23.61 R8.2 12.38,21.77 U3.3 | v5.08,34.29 v13.46,34.29 | J5.11 v3.81,26.67
  Bottom/Vert 0.127: v3.81,26.67 3.81,33.02 v5.08,34.29 | v13.46,34.29 13.46,25.05 12.99,24.58 12.99,24.09 v13.46,23.62
V_BATT
  Top/Horz 0.305: U4.3 6.6,27.68 6.48,27.56 6.1,27.56 | 6.1,27.56 4.94,27.56 4.45,27.06 4.45,24.16 | U4.2 6.1,27.56 | C15.1 7.4,22.93 U1.3
  Top/Horz 0.559: Q3.3 7.53,19.05 J4.2 7.12,18.92 C6.1 7.12,21.6 7.3,21.78 U1.3 7.3,23.66 6.81,24.16 4.45,24.16 1.29,24.16 J5.12
V_USB  (via drill 0.3)
  Top/Horz 0.432: J1.VBUS1 8.98,5.34 9.27,5.05 9.27,4.7 9.78,4.19 v9.93,4.19 13.13,4.19 13.59,4.65 13.59,5.08 13.88,5.37 J1.VBUS2
  Top/Horz 0.559: v6.35,25.4 7.27,25.4 | 7.27,25.4 U1.4 | v2.29,7.11 2.29,8.13 1.78,8.64 v1.78,9.14 | v10.38,26.16 10.08,25.87 C19.1 8.37,25.87 7.9,25.4 7.27,25.4 | 10.31,18.1 v10.38,18.16 | Q3.1 10.31,18.1 | 10.31,18.1 10.28,18.07 D4.A 10.93,15.86 R7.2 | v4.45,29.21 J5.10
  Bottom/Vert 0.559: v4.45,29.21 4.45,27.3 v6.35,25.4 | JP2.2 10.38,28.6 v10.38,26.16 v10.38,18.16 4.19,18.16 3.05,17.02 3.05,15.24 1.78,13.97 v1.78,9.14 | v9.93,4.19 8.21,2.46 5.79,2.46 2.29,5.97 v2.29,7.11
VIN
  Top/Horz 0.305: 13.34,19.94 13.34,16.51 | D4.C 13.34,16.51 | R8.1 13.34,21.73 13.34,19.94 | 13.34,19.94 13.27,20 Q3.2 11.56,20 10.48,21.08 | U5.1 13.82,16.51 13.34,16.51 | U3.1 10.48,21.08 | C7.1 10.4,21.01 10.48,21.08

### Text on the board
Bottom/Vert: v40
tPlace: + | -
Measures: Units in inches
tDocu: Nathan Seidle | Revised by: | Alex Brudner

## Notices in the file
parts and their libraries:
SparkFun-Aesthetics: Licensing: Creative Commons ShareAlike 4.0 International - https://creativecommons.org/licenses/by-sa/4.0
SparkFun-Aesthetics: Released under the Creative Commons Attribution Share-Alike 4.0 License
SparkFun-Aesthetics: https://creativecommons.org/licenses/by-sa/4.0
